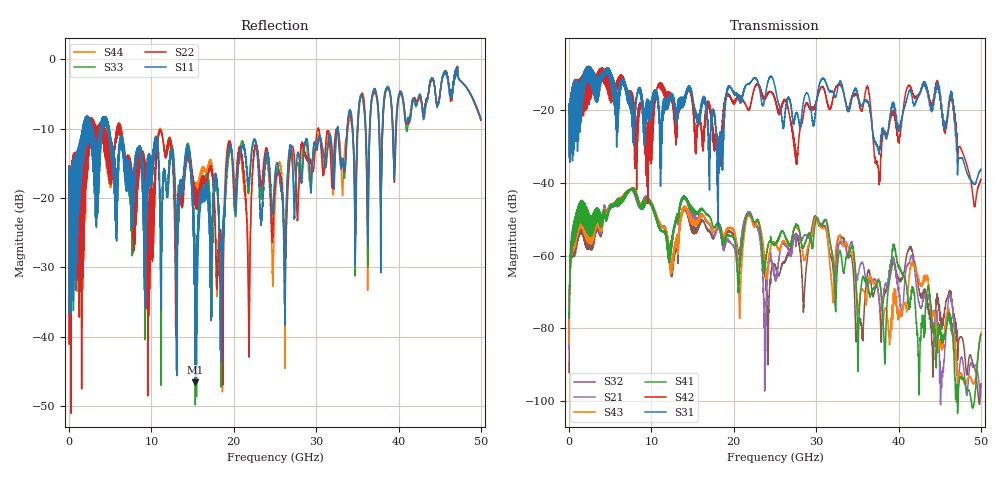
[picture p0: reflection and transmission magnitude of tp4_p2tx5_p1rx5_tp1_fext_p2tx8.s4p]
! 100G CR Analysis
! File: tp4_p2tx5_p1rx5_tp1_fext_p2tx8
! Description: 2m Cu Cable, OSFP, TP1-TP4
! Port Mapping
! Port1 -- P1RX5N
! Port2 -- P2TX8N
! Port3 -- P1RX5P
! Port4 -- P2TX8P
# GHz S MA R 50.00
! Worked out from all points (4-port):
!   5000 points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, 10 MHz to 50 GHz, reference 50 ohm
!   strongest paths, dB at 10 MHz, 12.51 GHz, 25.01 GHz, 37.51 GHz, 50 GHz:
!     S31: -20.6, -15.7, -13.7, -30.7, -36.3
!     S42: -20.5, -17.1, -16.9, -35.9, -39.0
!     S41: -75.7, -55.1, -57.0, -67.2, -81.7
!     S43: -84.2, -62.5, -56.3, -66.8, -81.2
!     S21: -85.6, -56.2, -66.2, -69.6, -97.7
!     S32: -92.1, -64.1, -62.5, -69.6, -95.2
!   lowest |S11| = -46.6 dB at 15.32 GHz (marker M1), VSWR 1.01, Z = 49.9 - j0.465 ohm
!   |S11| at or under -10 dB: start of sweep to 1.658 GHz; 4.861 GHz to 32.52 GHz (27.66 GHz wide, 148 % of centre); 32.66 GHz to 33.81 GHz (1.154 GHz wide, 3.47 % of centre)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
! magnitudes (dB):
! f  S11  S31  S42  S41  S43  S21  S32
! 10 MHz  -17.9  -20.6  -20.5  -75.7  -84.2  -85.6  -92.1
! 7.27 GHz  -18.8  -18.3  -17.7  -42.0  -41.9  -41.9  -42.0
! 15.32 GHz  -46.6  -21.0  -27.9  -48.5  -51.5  -50.3  -53.8
! 36.2 GHz  -17.2  -17.4  -13.4  -66.7  -69.7  -69.0  -65.2
! 37.56 GHz  -7.5  -30.1  -36.0  -66.8  -66.4  -70.3  -70.2
! 44.72 GHz  -6.7  -13.1  -12.3  -81.8  -83.6  -78.4  -71.8
! 50 GHz  -8.6  -36.3  -39.0  -81.7  -81.2  -97.7  -95.2
